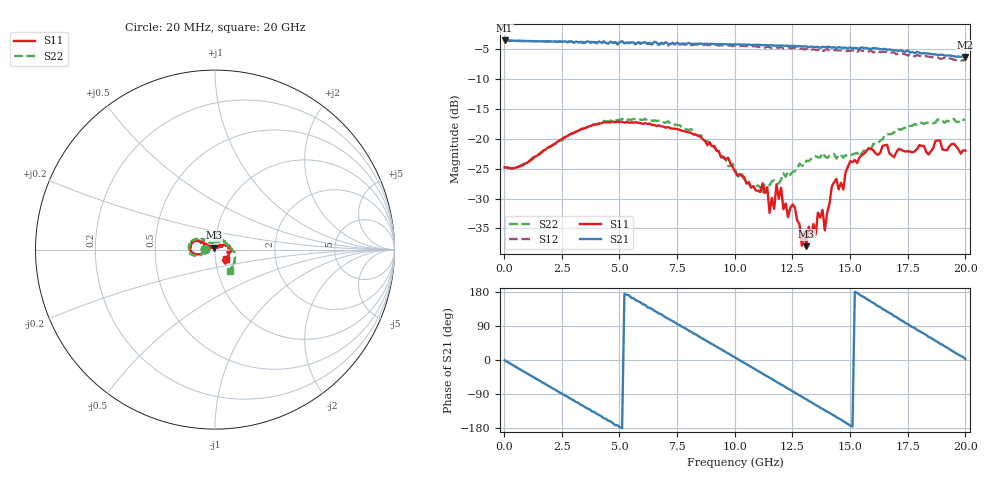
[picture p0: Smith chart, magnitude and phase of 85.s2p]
!Agilent Technologies,N5230A,US43500223,A.07.50.48
!Agilent N5230A: A.07.50.48
!Date: Thursday, October 08, 2015 16:13:49
!Correction: S11(Full 2 Port(1,2))
!S21(Full 2 Port(1,2))
!S12(Full 2 Port(1,2))
!S22(Full 2 Port(1,2))
!S2P File: Measurements: S11, S21, S12, S22:
# Hz S  RI  R 50
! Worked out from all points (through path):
!   201 points, 20 MHz to 20 GHz, reference 50 ohm
!   highest |S21| = -3.50 dB at 20 MHz (marker M1); lowest = -6.3 dB at 20 GHz (marker M2)
!   group delay of S21, straight-line fit = 99.3 ps
!   lowest |S11| = -38.0 dB at 13.11 GHz (marker M3), VSWR 1.03, Z = 49.5 + j1.15 ohm
!   |S11| at or under -10 dB: start of sweep to end of sweep
!   |S22| runs from -29.2 to -16.6 dB; largest |S21 - S12| = 0.061
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2e7  -0.0578 0.000835  0.6684 -0.00858  0.6689 -0.0098  -0.058 0.00149
1.9181e9  -0.0814 -0.0252  0.2441 -0.6132  0.2342 -0.6151  -0.0802 -0.0285
3.4166e9  -0.1198 -0.0205  -0.3294 -0.5595  -0.3324 -0.541  -0.1185 -0.0327
5.1149e9  -0.139 0.0148  -0.6608 -0.000706  -0.6503 0.0151  -0.1476 0.00131
6.7133e9  -0.1226 0.0438  -0.3315 0.5195  -0.3136 0.5272  -0.1365 0.0394
8.012e9  -0.101 0.052  0.139 0.6229  0.1572 0.6049  -0.1032 0.0595
1.001e10  -0.0472 0.025  0.6163 0.073  0.605 0.0443  -0.0321 0.0448
1.14086e10  -0.0353 0.0174  0.4455 -0.4163  0.4116 -0.4263  -0.0014 0.0402
1.15085e10  -0.0174 0.0165  0.4174 -0.4441  0.3784 -0.4483  0.0029 0.0407
1.2008e10  -0.0331 0.0207  0.2573 -0.5482  0.2269 -0.5469  0.0107 0.0443
1.21079e10  -0.02 0.0164  0.229 -0.5622  0.1819 -0.5428  0.0155 0.0491
1.26074e10  -0.0224 0.0143  0.0427 -0.601  0.00208 -0.581  0.0279 0.0459
1.31069e10  -0.00501 0.0116  -0.1403 -0.5781  -0.1577 -0.5444  0.0424 0.0503
1.34066e10  0.00137 0.0193  -0.2477 -0.535  -0.2607 -0.5008  0.0461 0.051
1.38062e10  0.0223 0.0122  -0.3718 -0.4605  -0.3662 -0.4055  0.0601 0.0472
1.39061e10  0.0126 0.0117  -0.3996 -0.4304  -0.3894 -0.3916  0.0585 0.0414
1.42058e10  0.0293 0.0271  -0.4671 -0.347  -0.4578 -0.32  0.0647 0.0343
1.47053e10  0.0313 0.0211  -0.5519 -0.1824  -0.5292 -0.1484  0.0633 0.0288
1.5005e10  0.0613 0.0217  -0.5809 -0.073  -0.5425 -0.0622  0.0701 0.0199
1.67033e10  0.0744 -0.0147  -0.3136 0.4652  -0.2798 0.4415  0.1075 -0.021
1.83017e10  0.0518 -0.0585  0.2109 0.4769  0.2307 0.4377  0.0984 -0.0941
2e10  0.0589 -0.0538  0.4856 0.024  0.4558 -0.00719  0.083 -0.1188
